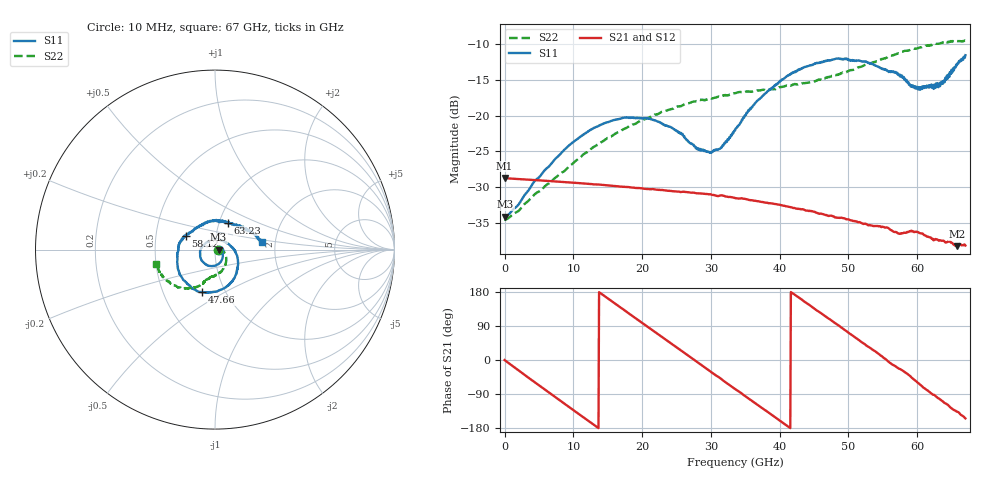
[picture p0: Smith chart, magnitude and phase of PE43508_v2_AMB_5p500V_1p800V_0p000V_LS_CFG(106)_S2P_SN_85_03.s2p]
!Keysight Technologies,N5227A,US51270237,A.10.43.00
!Date: Wednesday, August 22, 2018 17:17:44
!Correction: S11(Full 2 Port(1,3))
!S31(Full 2 Port(1,3))
!S13(Full 2 Port(1,3))
!S33(Full 2 Port(1,3))
!S2P File: Measurements: S11, S31, S13, S33:
# Hz S  dB  R 50
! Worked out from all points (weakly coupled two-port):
!   801 points, 10 MHz to 67 GHz, reference 50 ohm
!   highest |S21| = -28.74 dB at 10 MHz (marker M1); lowest = -38.3 dB at 65.83 GHz (marker M2)
!   lowest |S11| = -34.2 dB at 93.74 MHz (marker M3), VSWR 1.04, Z = 52 + j0.00665 ohm
!   |S11| at or under -10 dB: start of sweep to end of sweep
!   |S22| runs from -34.6 to -9.4 dB; largest |S21 - S12| = 0.00021
!   S11 on the Smith chart (normalised r, x): 10 MHz: 1.04, -0.00; 47.66 GHz: 0.78, -0.39; 58.12 GHz: 0.71, +0.11; 63.23 GHz: 1.10, +0.34; 67 GHz: 1.71, +0.15
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1e7  -34.09 -1.0  -28.74 -0.3  -28.74 -0.2  -34.53 -0.6
9.37375e7  -34.16 0.2  -28.75 -1.4  -28.76 -1.4  -34.58 0.6
7.462638e9  -25.97 -31.0  -29.22 -99.1  -29.22 -99.1  -28.64 -0.3
1.123082e10  -22.78 -61.5  -29.48 -148.3  -29.48 -148.2  -25.63 -15.0
1.74274e10  -20.27 -111.6  -29.96 131.4  -29.96 131.4  -21.81 -39.0
2.236791e10  -20.83 -154.6  -30.39 67.5  -30.39 67.5  -19.71 -57.3
2.580115e10  -22.63 168.2  -30.67 23.6  -30.66 23.6  -18.57 -68.3
2.797832e10  -24.54 131.6  -30.87 -4.7  -30.87 -4.8  -17.95 -74.2
2.973681e10  -25.12 97.3  -31.01 -27.6  -31.00 -27.6  -17.58 -79.1
3.132782e10  -24.61 64.1  -31.19 -47.6  -31.19 -47.7  -17.28 -83.6
3.3505e10  -22.07 24.5  -31.52 -76.5  -31.52 -76.6  -16.83 -89.1
3.836178e10  -16.50 -30.8  -32.25 -138.5  -32.26 -138.4  -16.39 -97.5
4.15438e10  -14.21 -58.8  -32.82 -179.7  -32.82 -179.7  -15.75 -101.4
4.472582e10  -12.87 -83.7  -33.39 139.7  -33.39 139.8  -15.27 -105.2
4.765664e10  -12.14 -106.5  -34.06 102.2  -34.05 102.1  -14.41 -108.9
5.234594e10  -12.38 -144.0  -35.14 42.1  -35.11 42.0  -12.90 -114.9
5.586291e10  -13.86 -179.4  -35.80 -5.3  -35.79 -5.6  -11.68 -124.1
5.812382e10  -14.93 155.1  -36.41 -31.1  -36.40 -31.5  -10.93 -130.6
6.004979e10  -15.95 122.2  -36.29 -59.3  -36.29 -59.6  -10.55 -137.4
6.323181e10  -15.52 64.3  -37.45 -102.7  -37.51 -103.2  -9.87 -150.0
6.582768e10  -12.72 24.0  -38.29 -136.5  -38.38 -136.9  -9.54 -159.8
6.7e10  -11.50 8.7  -38.21 -154.0  -38.29 -154.1  -9.46 -166.0
